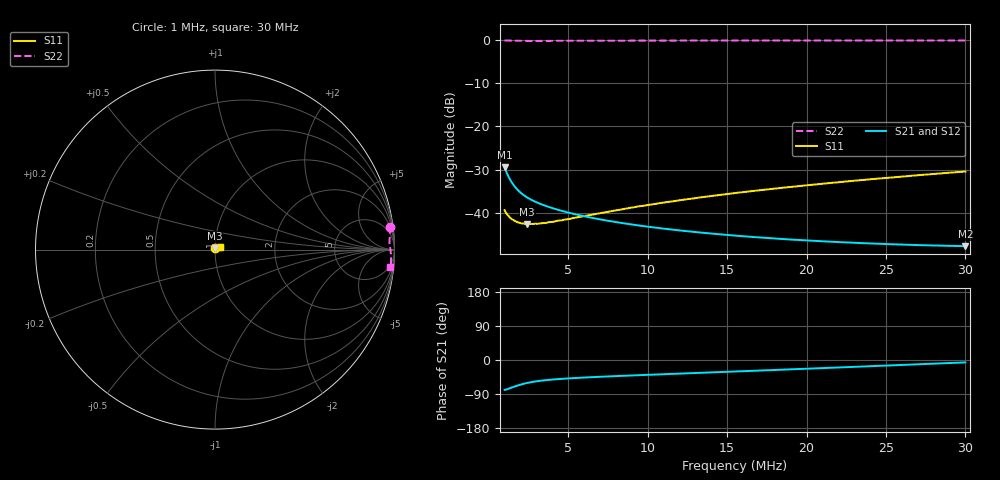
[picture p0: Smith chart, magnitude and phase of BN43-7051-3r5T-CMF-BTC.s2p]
! ListType=Log
!!BN43-7051 3.5T CMF Barrel Thru Cal
# MHZ S RI R 50
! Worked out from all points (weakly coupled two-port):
!   101 points, 1 MHz to 30 MHz, reference 50 ohm
!   highest |S21| = -29.51 dB at 1 MHz (marker M1); lowest = -47.7 dB at 30 MHz (marker M2)
!   lowest |S11| = -42.6 dB at 2.421 MHz (marker M3), VSWR 1.01, Z = 49.9 + j0.728 ohm
!   |S11| at or under -10 dB: start of sweep to end of sweep
!   |S22| runs from -0.2 to -0.1 dB; largest |S21 - S12| = 0.0001
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1  -0.00221 0.0105  0.00649 -0.0328  0.00653 -0.0327  0.9756 0.1282
1.107423  -0.00204 0.00967  0.00635 -0.0291  0.0064 -0.0291  0.9761 0.113
1.312713  -0.0019 0.00867  0.00652 -0.024  0.00656 -0.0239  0.9754 0.0918
1.453729  -0.00184 0.00827  0.00671 -0.0214  0.00675 -0.0214  0.9747 0.0812
1.609893  -0.00177 0.00795  0.00691 -0.0193  0.00693 -0.0192  0.974 0.072
1.844513  -0.00169 0.00756  0.00713 -0.0168  0.00714 -0.0168  0.9731 0.0614
1.97435  -0.00153 0.00751  0.00722 -0.0158  0.00723 -0.0157  0.9727 0.0567
2.042657  -0.00145 0.00743  0.00725 -0.0153  0.00726 -0.0153  0.9726 0.0545
2.421316  -0.00127 0.0073  0.00739 -0.0131  0.00739 -0.0131  0.9721 0.0448
2.969469  -0.000821 0.00746  0.00737 -0.0111  0.00737 -0.0111  0.9721 0.0349
3.072204  -0.00075 0.00741  0.00735 -0.0108  0.00734 -0.0108  0.9721 0.0334
3.89806  -7.84e-05 0.00782  0.00708 -0.00907  0.00707 -0.00908  0.9732 0.0237
4.780527  0.000603 0.00834  0.00674 -0.00782  0.00674 -0.00783  0.9745 0.0158
5.862773  0.00148 0.00893  0.00636 -0.00673  0.00635 -0.00675  0.976 0.00772
7.9624  0.0032 0.0102  0.00577 -0.00531  0.00576 -0.00534  0.978 -0.00492
9.438436  0.0045 0.011  0.00547 -0.0046  0.00545 -0.00464  0.9791 -0.0126
10.81396  0.00572 0.0117  0.00524 -0.00407  0.00521 -0.00411  0.9797 -0.0192
13.2621  0.00798 0.0127  0.00492 -0.00331  0.0049 -0.00335  0.9805 -0.0304
15.72057  0.0105 0.0136  0.00469 -0.0027  0.00467 -0.00276  0.9808 -0.0409
20.63659  0.0158 0.0144  0.00438 -0.00177  0.00434 -0.00184  0.9805 -0.0607
25.30843  0.0214 0.014  0.0042 -0.00107  0.00415 -0.00114  0.9794 -0.0788
30  0.0274 0.0124  0.00409 -0.000452  0.00403 -0.000534  0.9777 -0.0965
